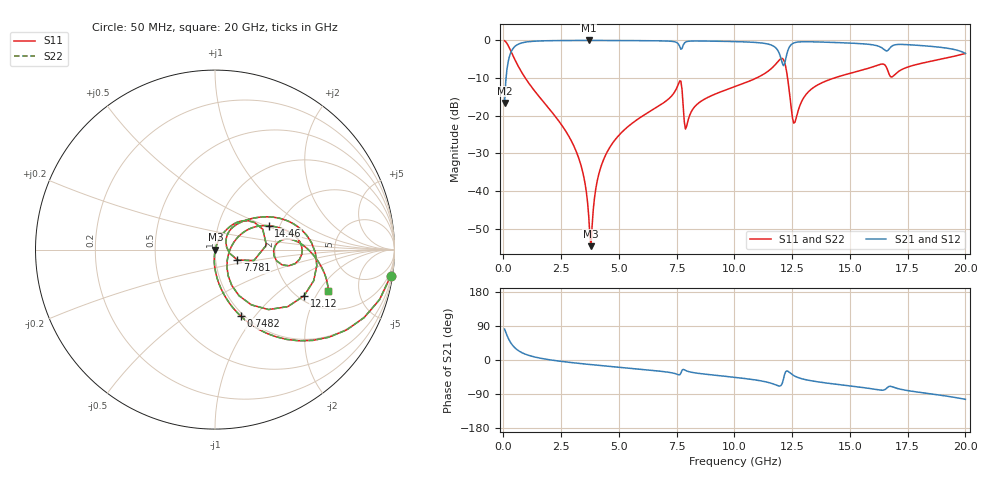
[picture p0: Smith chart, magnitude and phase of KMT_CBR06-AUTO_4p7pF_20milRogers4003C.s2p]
! Data measured by Modelithics Inc. support@modelithics.com 813-866-6335
! KEMET CBR06-AUTO 4.7pF, Pad Width= 0.851mm, Pad Length= 0.64mm, Pad Gap= 0.62mm, 20mil Rogers 4003C substrate Data, January 2022
# hz S ma R 50
! 2 Port Network Data from SP1.SP block
! freq  magS11  angS11  magS21  angS21  magS12  angS12  magS22  angS22
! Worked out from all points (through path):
!   401 points, 50 MHz to 20 GHz, reference 50 ohm
!   highest |S21| = -0.02 dB at 3.691 GHz (marker M1); lowest = -16.6 dB at 50 MHz (marker M2)
!   group delay of S21, straight-line fit = 15.8 ps
!   lowest |S11| = -54.6 dB at 3.791 GHz (marker M3), VSWR 1.00, Z = 50.2 + j0.0206 ohm
!   |S11| at or under -10 dB: 946.4 MHz to 10.95 GHz (10 GHz wide, 168 % of centre); 12.3 GHz to 14.31 GHz (2.013 GHz wide, 15.1 % of centre)
!   |S22| runs from -54.6 to -0.1 dB; largest |S21 - S12| = 0
!   S11 on the Smith chart (normalised r, x): 50 MHz: 1, -13; 748.2 MHz: 0.97, -0.85; 7.781 GHz: 1.28, -0.15; 12.12 GHz: 2.15, -1.61; 14.46 GHz: 1.75, +0.52; 20 GHz: 2.91, -2.43
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5e7  0.9891 -8.6  0.1472 81.4  0.1472 81.4  0.9891 -8.6
2.99375e8  0.7442 -42.8  0.6671 47.1  0.6671 47.1  0.7442 -42.8
7.4825e8  0.3964 -68.9  0.9171 21.0  0.9171 21.0  0.3964 -68.9
2.693375e9  0.06261 -93.7  0.9964 -5.0  0.9964 -5.0  0.06261 -93.7
3.391625e9  0.02002 -94.9  0.998 -9.7  0.998 -9.7  0.02002 -94.9
3.690875e9  0.004697 -79.9  0.9981 -11.6  0.9981 -11.6  0.004697 -79.9
3.790625e9  0.001852 6.4  0.9981 -12.2  0.9981 -12.2  0.001852 6.4
4.089875e9  0.01499 69.1  0.9979 -13.9  0.9979 -13.9  0.01499 69.1
4.53875e9  0.03516 70.3  0.9973 -16.5  0.9973 -16.5  0.03516 70.3
6.73325e9  0.1351 59.2  0.9869 -29.2  0.9869 -29.2  0.1351 59.2
7.581125e9  0.2669 34.4  0.89 -38.9  0.89 -38.9  0.2669 34.4
7.780625e9  0.1379 -24.9  0.8618 -24.7  0.8618 -24.7  0.1379 -24.9
7.93025e9  0.07242 32.4  0.9629 -28.9  0.9629 -28.9  0.07242 32.4
1.0025e10  0.2438 42.9  0.9641 -45.9  0.9641 -45.9  0.2438 42.9
1.167088e10  0.4434 20.5  0.8465 -63.0  0.8465 -63.0  0.4434 20.5
1.211975e10  0.559 -27.4  0.4623 -51.2  0.4623 -51.2  0.559 -27.4
1.256862e10  0.07978 -22.5  0.9236 -41.0  0.9236 -41.0  0.07978 -22.5
1.336662e10  0.2298 30.9  0.9574 -55.3  0.9574 -55.3  0.2298 30.9
1.446388e10  0.3272 24.0  0.9354 -64.4  0.9354 -64.4  0.3272 24.0
1.670825e10  0.3491 -10.4  0.7746 -69.5  0.7746 -69.5  0.3491 -10.4
1.775562e10  0.4674 5.0  0.8678 -83.1  0.8678 -83.1  0.4674 5.0
2e10  0.6713 -20.0  0.6712 -103.8  0.6712 -103.8  0.6713 -20.0
